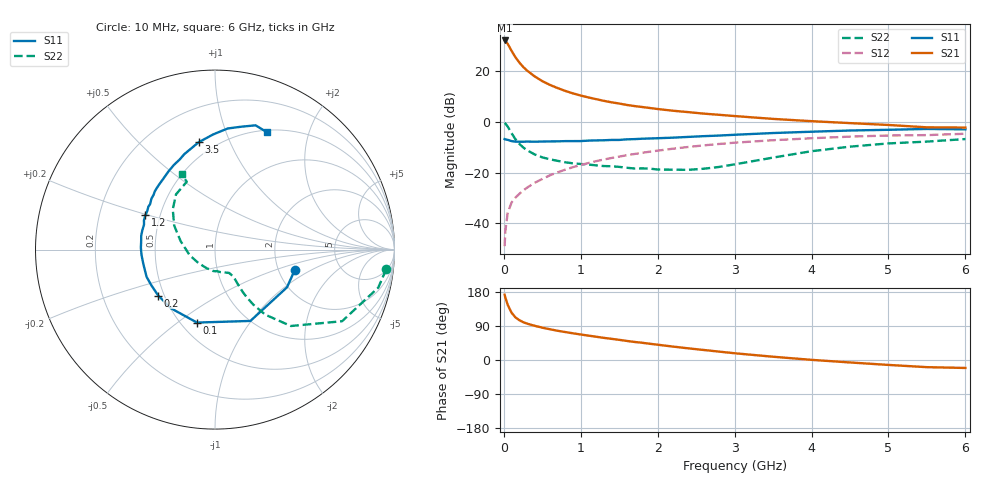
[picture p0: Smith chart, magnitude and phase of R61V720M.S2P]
! SIEMENS Small Signal Semiconductors
! BFR193
! Si NPN RF Bipolar Junction Transistor in SOT23
! VCE = 1.75 V  IC = 20 mA
! Common Emitter S-Parameters:  May  1996
# GHz  S  MA  R  50
!  f  S11  S21  S12  S22
! GHz  MAG  ANG  MAG  ANG  MAG  ANG  MAG  ANG
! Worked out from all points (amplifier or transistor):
!   36 points, 10 MHz to 6 GHz, reference 50 ohm
!   highest |S21| = 32.2 dB at 10 MHz (marker M1)
!   |S21| within 3 dB of that: start of sweep to 80.23 MHz
!   unconditionally stable (mu >= 1): 521.7 MHz to 1.894 GHz
!   at 250 MHz: K = 0.84, MSG = 24.5 dB, |S12| = -27.2 dB
!   at 1.4 GHz: K = 1.03, MAG = 10.0 dB, |S12| = -14.2 dB
!   at 6 GHz: K = 0.95, MSG = 1.2 dB, |S12| = -4.6 dB
!   S11 on the Smith chart (normalised r, x): 10 MHz: 2.46, -0.71; 100 MHz: 0.60, -0.59; 200 MHz: 0.46, -0.29; 1.2 GHz: 0.41, +0.20; 3.5 GHz: 0.41, +0.77; 6 GHz: 0.52, +1.40
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0.01  0.4589 -14.3  40.97 172.3  0.0035 85.1  0.9599 -6.6
0.02  0.4528 -27.7  40.15 164.7  0.0071 77.0  0.934 -13.1
0.05  0.4437 -63.6  35.11 145.6  0.0159 69.3  0.8129 -29.4
0.1  0.4188 -103.9  25.59 125.0  0.0255 61.5  0.5999 -45.2
0.15  0.4088 -127.0  19.15 112.6  0.0319 61.3  0.4583 -52.3
0.2  0.407 -140.9  15.11 105.3  0.0377 62.6  0.372 -55.2
0.25  0.4067 -150.9  12.32 100.0  0.0439 63.8  0.3151 -56.4
0.3  0.4103 -158.3  10.45 96.1  0.05 65.3  0.2774 -56.8
0.4  0.4072 -168.7  7.987 90.3  0.0626 67.0  0.2286 -56.5
0.5  0.4105 -175.8  6.425 85.3  0.0748 68.3  0.1997 -56.0
0.6  0.4131 178.5  5.408 81.1  0.0883 68.4  0.1825 -56.1
0.7  0.4142 173.3  4.676 77.1  0.1012 68.4  0.1703 -56.9
0.8  0.4185 169.1  4.106 73.7  0.1143 67.8  0.1596 -57.9
0.9  0.4189 164.9  3.673 70.4  0.1281 67.3  0.152 -58.9
1.1  0.4284 157.5  3.055 64.3  0.1544 65.5  0.1439 -63.7
1.2  0.4323 153.7  2.829 61.4  0.1681 64.4  0.1387 -66.4
1.6  0.4539 141.3  2.171 50.3  0.2201 59.7  0.1244 -80.7
2.2  0.4898 125.7  1.668 35.4  0.2965 51.5  0.114 -112.7
3.5  0.6047 98.7  1.151 8.6  0.4359 31.3  0.1977 166.0
4.5  0.6786 84.0  0.95 -6.5  0.5136 17.0  0.3254 136.3
5.5  0.7285 71.9  0.784 -18.9  0.5504 2.7  0.4094 112.6
6  0.7152 66.3  0.776 -21.0  0.5858 -1.5  0.4596 113.8
